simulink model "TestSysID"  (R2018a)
settings: Solver=FixedStepAuto  StartTime=0.0  StopTime=10.0  FixedStep=0.1  RelTol=1e-3

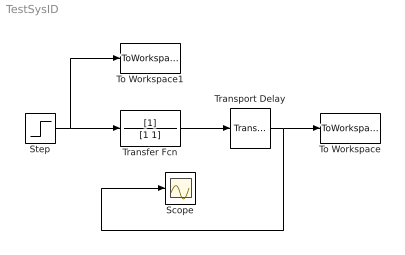
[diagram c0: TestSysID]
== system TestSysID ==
  Scope : Scope
  Step : Step  SampleTime=0
  To Workspace : ToWorkspace  VariableName=yout  SampleTime=-1
  To Workspace1 : ToWorkspace  VariableName=uout  SampleTime=-1
  Transfer Fcn : TransferFcn  Denominator=[1 1]
  Transport Delay : TransportDelay  DelayTime=3
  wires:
  Step/1 -> To Workspace1/1, Transfer Fcn/1
  Transfer Fcn/1 -> Transport Delay/1
  Transport Delay/1 -> Scope/1, To Workspace/1
